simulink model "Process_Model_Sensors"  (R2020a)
settings: Solver=ode45  StartTime=0.0  StopTime=480000  RelTol=1e-3  EnableMultiTasking=on
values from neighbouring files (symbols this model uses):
  C = V*rho_a*c_a    (= 62550.8352)    [balloon_init.m]
  f = 1.2000    (= 1.2)    [balloon_init.m]
  g = 9.80665    [balloon_init.m]
  K = 1.0e+03 * [1.1698    0.0100    0.0993]    [balloon_init.m]
  m = 12    [balloon_init.m]
  rho_a = 1.2928    [balloon_init.m]
  Ta = 20+273.15    (= 293.15)    [balloon_init.m]
  theta_t = 0.0800    (= 0.08)    [balloon_init.m]
  Ts = 8    [balloon_init.m]    (also in train_net.m)
  V = 48    [balloon_init.m]
  x1_0 = x1_d    (= 363.429535865)    [balloon_init.m]
  x2_0 = 100    [balloon_init.m]
  x2_d = 120    [balloon_init.m]
  x3_0 = 0    [balloon_init.m]
  x3_d = 0    [balloon_init.m]

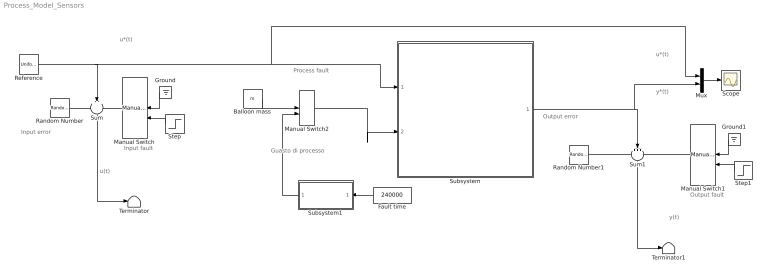
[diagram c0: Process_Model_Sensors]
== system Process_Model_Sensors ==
  note: Process fault
  note: u(t)
  note: Input fault
  note: Input error
  note: u*(t)
  note: y*(t)
  note: u*(t)
  note: Output error
  note: Output fault
  note: y(t)
  note: Guasto di processo
  Balloon mass : Constant  Value=m
  Fault time : Constant  Value=240000
  Ground : Ground
  Ground1 : Ground
  Manual Switch : ManualSwitch
  Manual Switch1 : ManualSwitch
  Manual Switch2 : ManualSwitch
  Mux : Mux  Inputs=2
  Random Number : RandomNumber  Variance=0.05  Seed=2  SampleTime=Ts
  Random Number1 : RandomNumber  Variance=0.05  Seed=3  SampleTime=Ts
  Reference : UniformRandomNumber  Minimum=x2_d*0.9  Maximum=x2_d*1.1  Seed=1  SampleTime=800
  Scope : Scope
  Step : Step  Time=240000  After=10  SampleTime=0
  Step1 : Step  Time=240000  After=10  SampleTime=0
  Subsystem : Subsystem
  Subsystem1 : Subsystem
  Sum : Sum  Inputs=+++
  Sum1 : Sum  Inputs=+++
  Terminator : Terminator
  Terminator1 : Terminator
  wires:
  Reference/1 -> Mux/1, Subsystem/1(u*), Sum/2
  Mux/1 -> Scope/1
  Random Number/1 -> Sum/1
  Manual Switch/1 -> Sum/3
  Sum/1 -> Terminator/1
  Ground/1 -> Manual Switch/1
  Step/1 -> Manual Switch/2
  Sum1/1 -> Terminator1/1
  Step1/1 -> Manual Switch1/2
  Random Number1/1 -> Sum1/1
  Subsystem/1(y*) -> Mux/2, Sum1/2
  Ground1/1 -> Manual Switch1/1
  Manual Switch1/1 -> Sum1/3
  Fault time/1 -> Subsystem1/1(Fault time)
  Subsystem1/1(Fault) -> Manual Switch2/2
  Manual Switch2/1 -> Subsystem/2(m)
  Balloon mass/1 -> Manual Switch2/1

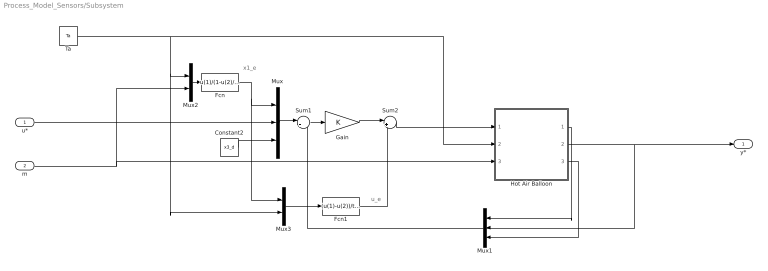
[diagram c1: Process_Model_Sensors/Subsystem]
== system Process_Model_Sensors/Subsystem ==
  note: x1_e
  note: u_e
  u* : Inport
  m : Inport  Port=2
  Constant2 : Constant  Value=x3_d
  Fcn : Fcn  Expr=u(1)/(1-u(2)/(V*rho_a))
  Fcn1 : Fcn  Expr=(u(1)-u(2))/theta_t
  Gain : Gain  Gain=K  Multiplication=Matrix(K*u)  SaturateOnIntegerOverflow=on
  Hot Air Balloon : Subsystem  mask{V=V, m=m, C=C, theta_t=theta_t, f=f, g=g}
      mask prompts: V "Balloon's volume (V)"; m "Balloon's total mass (m)"; C "Thermal capacitance (C)"; theta_t "Thermal resistance (theta_t)"; f "Aerodynamic viscous friction (f)"; g "Gravitational acceleration (g)"
  Mux : Mux  Inputs=3
  Mux1 : Mux  Inputs=3
  Mux2 : Mux  Inputs=2
  Mux3 : Mux  Inputs=2
  Sum1 : Sum  Inputs=|+-  InputSameDT=on  SaturateOnIntegerOverflow=on
  Sum2 : Sum  Inputs=|++  InputSameDT=on  SaturateOnIntegerOverflow=on
  Ta : Constant  Value=Ta
  y* : Outport
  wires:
  Ta/1 -> Mux2/1, Mux3/2, Hot Air Balloon/2(Ta)
  Hot Air Balloon/2(x2) -> y*/1, Mux1/2
  Fcn1/1 -> Sum2/2
  Mux1/1 -> Sum1/2
  Hot Air Balloon/3(x3) -> Mux1/3
  Mux3/1 -> Fcn1/1
  Fcn/1 -> Mux/1, Mux3/1
  Gain/1 -> Sum2/1
  Sum2/1 -> Hot Air Balloon/1(u)
  Mux/1 -> Sum1/1
  Hot Air Balloon/1(x1) -> Mux1/1
  m/1 -> Mux2/2, Hot Air Balloon/3(m)
  Constant2/1 -> Mux/3
  u*/1 -> Mux/2
  Sum1/1 -> Gain/1
  Mux2/1 -> Fcn/1

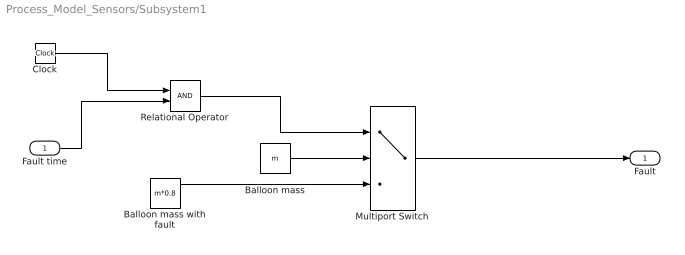
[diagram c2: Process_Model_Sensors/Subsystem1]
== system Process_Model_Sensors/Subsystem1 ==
  Fault time : Inport
  Balloon mass : Constant  Value=m
  Balloon mass with fault : Constant  Value=m*0.8
  Clock : Clock
  Multiport Switch : MultiPortSwitch  DataPortOrder=Zero-based contiguous  Inputs=2  zeroidx=on
  Relational Operator : RelationalOperator  OutDataTypeStr=boolean  RndMeth=Simplest
  Fault : Outport
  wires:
  Clock/1 -> Relational Operator/1
  Fault time/1 -> Relational Operator/2
  Balloon mass/1 -> Multiport Switch/2
  Relational Operator/1 -> Multiport Switch/1
  Multiport Switch/1 -> Fault/1
  Balloon mass with fault/1 -> Multiport Switch/3

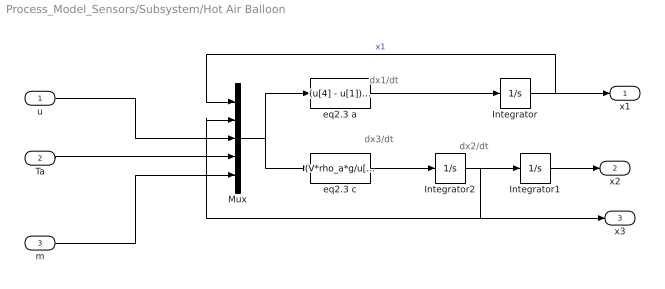
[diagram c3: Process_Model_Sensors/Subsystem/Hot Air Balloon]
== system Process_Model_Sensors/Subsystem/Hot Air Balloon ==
  note: dx2/dt
  note: dx3/dt
  note: dx1/dt
  u : Inport
  Ta : Inport  Port=2
  m : Inport  Port=3
  Integrator : Integrator  InitialCondition=x1_0
  Integrator1 : Integrator  InitialCondition=x2_0  LowerSaturationLimit=0
  Integrator2 : Integrator  InitialCondition=x3_0
  Mux : Mux  Inputs=5
  eq2.3 a : Fcn  Expr=(u[4] - u[1])/(C*theta_t) + u[3]/C
  eq2.3 c : Fcn  Expr=(V*rho_a*g/u[5])*(1 - u[4]/u[1]) - (f/u[5])*u[2] - g
  x1 : Outport
  x2 : Outport  Port=2
  x3 : Outport  Port=3
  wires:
  Ta/1 -> Mux/4
  u/1 -> Mux/3
  Integrator1/1 -> x2/1
  Integrator2/1 -> Mux/2, x3/1, Integrator1/1
  Integrator/1 -> x1/1, Mux/1  "x1"
  Mux/1 -> eq2.3 c/1, eq2.3 a/1
  eq2.3 c/1 -> Integrator2/1
  eq2.3 a/1 -> Integrator/1
  m/1 -> Mux/5
